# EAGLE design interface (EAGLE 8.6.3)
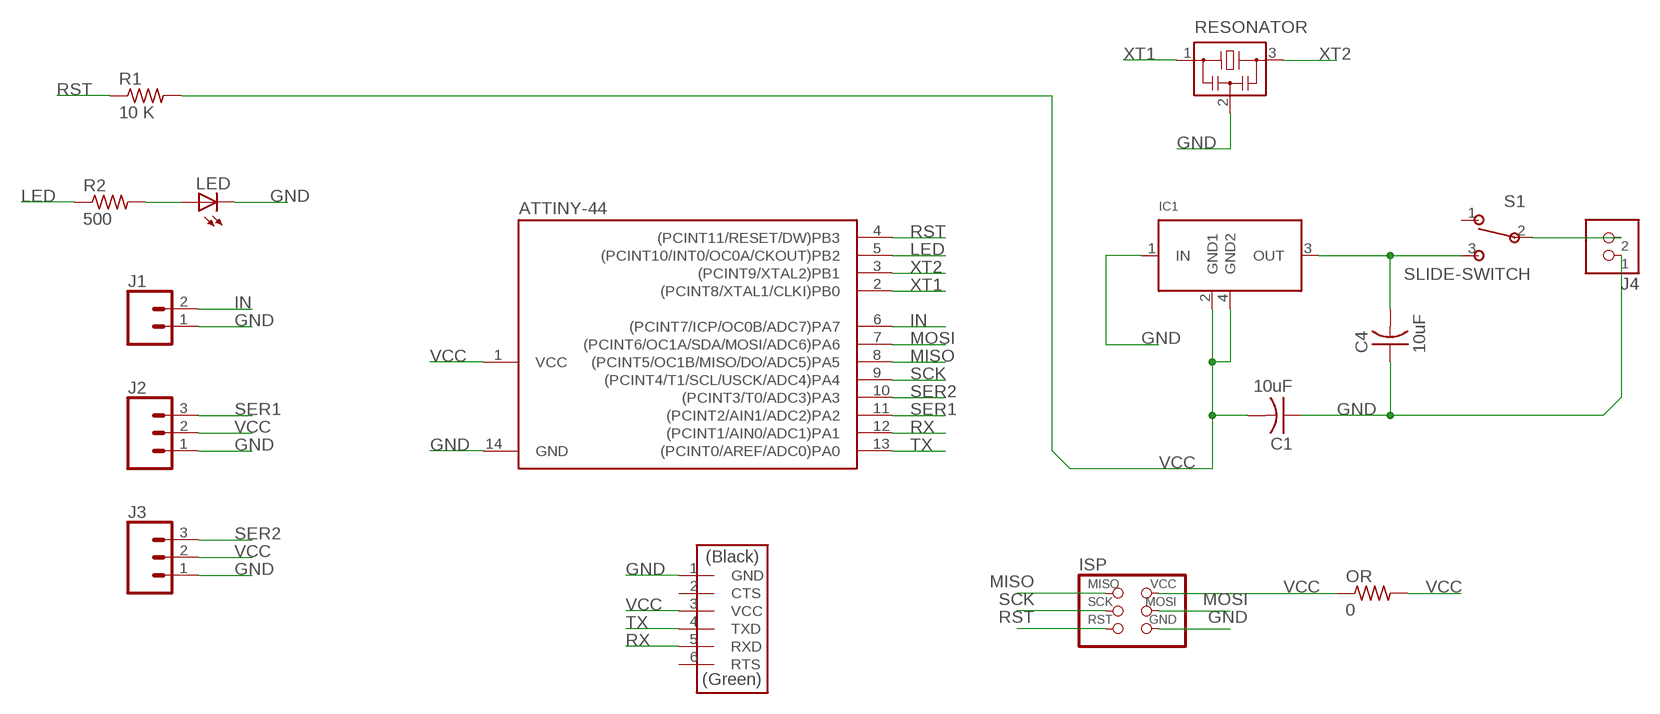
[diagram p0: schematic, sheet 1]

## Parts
ATTINY-44  ATTINY44-SSU  [SOIC14]
C1  10uF  CAP-US1206FAB  [C1206FAB]
C4  10uF  CAP-US1206FAB  [C1206FAB]
IC1  VREG_MULTI  [SOT223]
ISP  AVRISPSMD  [2X03SMD]
J1  CONN_02  [1X02]
J2  CONN_03  [1X03]
J3  CONN_03  [1X03]
J4  TERM-1X02-FABLAB  [ED555DS-2DS]
LED  LEDFAB1206  [LED1206FAB]
OR  0  RES-US1206FAB  [R1206FAB]
R1  10 K  RES-US1206FAB  [R1206FAB]
R2  500  RES-US1206FAB  [R1206FAB]
RESONATOR  RESONATOR  [EFOBM]
S1  SLIDE-SWITCH  [AYZ0102AGRLC]
U$1  FTDI-SMD-HEADER  [1X06SMD]

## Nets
GND: ATTINY-44.14(GND) C1.1 C4.1 IC1.1(IN) ISP.6(GND) J1.1 J2.1 J3.1 J4.1 LED.2(C) RESONATOR.2 U$1.1(GND)
IN: ATTINY-44.6((PCINT7/ICP/OC0B/ADC7)PA7) J1.2
LED: ATTINY-44.5((PCINT10/INT0/OC0A/CKOUT)PB2) R2.1
MISO: ATTINY-44.8((PCINT5/OC1B/MISO/DO/ADC5)PA5) ISP.1(MISO)
MOSI: ATTINY-44.7((PCINT6/OC1A/SDA/MOSI/ADC6)PA6) ISP.4(MOSI)
N$3: C4.2 IC1.3(OUT) S1.3
N$5: J4.2 S1.2
N$6: LED.1(A) R2.2
RST: ATTINY-44.4((PCINT11/RESET/DW)PB3) ISP.5(RST) R1.1
RX: ATTINY-44.12((PCINT1/AIN0/ADC1)PA1) U$1.5(RXD)
SCK: ATTINY-44.9((PCINT4/T1/SCL/USCK/ADC4)PA4) ISP.3(SCK)
SER1: ATTINY-44.11((PCINT2/AIN1/ADC2)PA2) J2.3
SER2: ATTINY-44.10((PCINT3/T0/ADC3)PA3) J3.3
TX: ATTINY-44.13((PCINT0/AREF/ADC0)PA0) U$1.4(TXD)
VCC: ATTINY-44.1(VCC) C1.2 IC1.2(GND1) IC1.4(GND2) ISP.2(VCC) J2.2 J3.2 OR.1 OR.2 R1.2 U$1.3(VCC)
XT1: ATTINY-44.2((PCINT8/XTAL1/CLKI)PB0) RESONATOR.1
XT2: ATTINY-44.3((PCINT9/XTAL2)PB1) RESONATOR.3
Unconnected: S1.1 U$1.2(CTS) U$1.6(RTS)

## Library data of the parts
ATTINY-44 = fab:ATTINY44
C1 C4 = fab:CAP-US
IC1 = m-pad-2.1:VREG_MULTI: standard package voltage regulator (LM2940, LM2937, LM340, UA78M05, etc)
ISP = fab:AVRISP
J1 = SparkFun-Connectors:CONN_02: Multi connection point. Often used as Generic Header-pin footprint for 0.1 inch spaced/style header connections
J2 J3 = SparkFun-Connectors:CONN_03: Multi connection point. Often used as Generic Header-pin footprint for 0.1 inch spaced/style header connections On any of the 0.1 inch spaced packages, you can populate with these: Break Away Headers - Straight (PRT-00116) Break Away Male Headers - Right Angle (PRT-00553) Female Headers (PRT-00115)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; PROD_ID: XXX-00000; VALUE: 455-1750-1-ND
J4 = fab:TERM-1X02: 3.5mm terminal block, 2 positions ED555-2DS as found in the fablab inventory.
LED = fab:LED: LED
OR R1 R2 = fab:RES-US: Resistor (US Symbol)
RESONATOR = fab:RESONATOR
S1 = fab:SLIDE-SWITCH: SMD slide-switch AYZ0102AGRLC as found in the fablab inventory. Includes the mounting holes. Made by Zaerc.
U$1 = fab:FTDI-SMD-HEADER

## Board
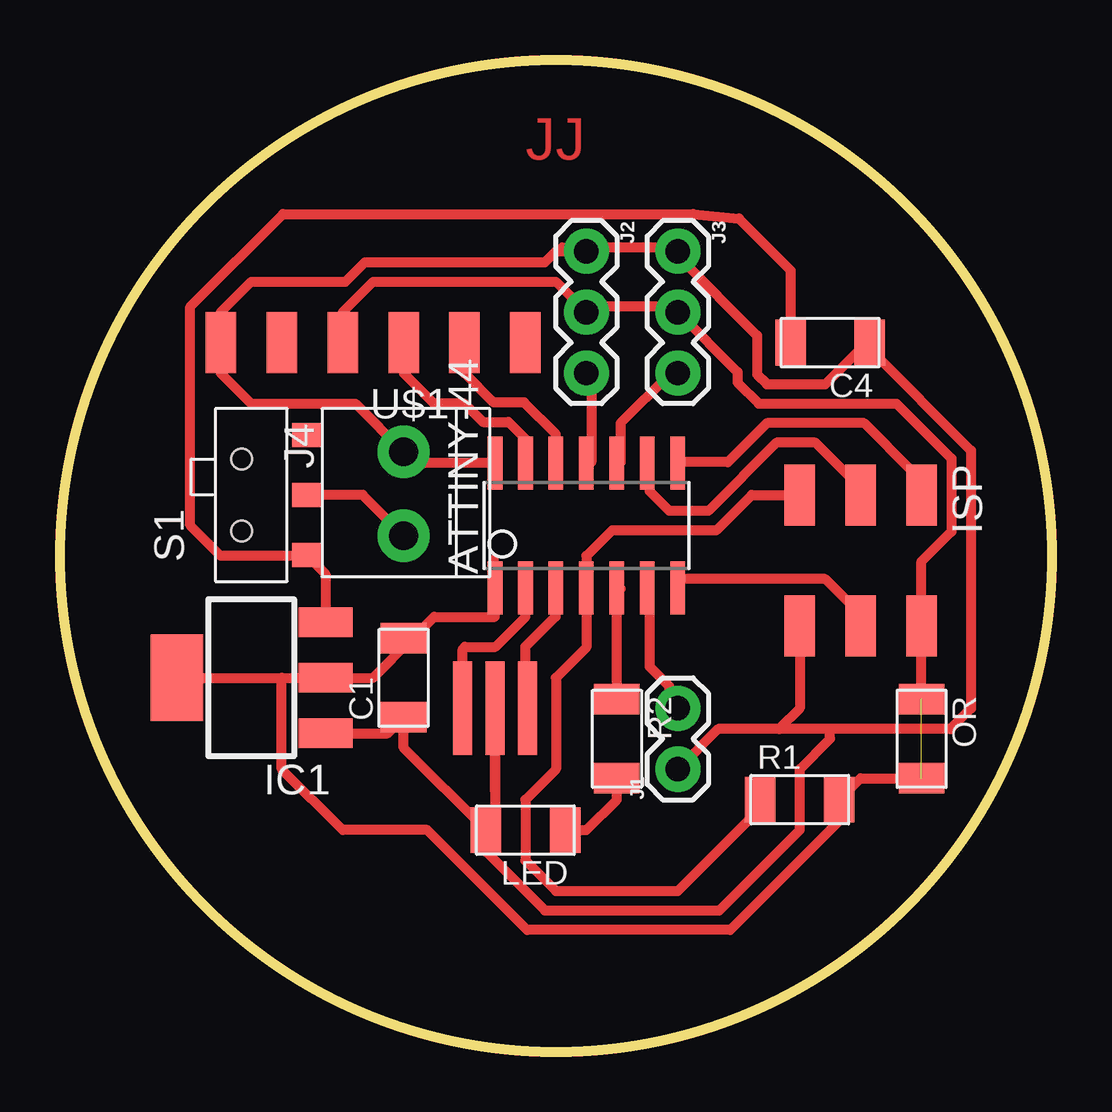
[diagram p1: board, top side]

Size 41.35 x 41.35 mm. Coordinates in mm from the lower left corner, seen from the top.
Outline: circle at 20.67,20.67 radius 20.67
Copper layers (1*16): Top 0.035mm / dielectric 1.5mm / Bottom 0.035mm
Design rules "default *": minimum track width 16mil, minimum drill 0.35mm, track to track 16mil, track to pad 16mil, pad to pad 16mil, via to via 16mil, smd to smd 16mil, copper to edge 16mil, drill to drill 16mil, minimum pad ring 10mil, minimum via ring 8mil, stop-mask expansion 4mil, vias tented up to drill 0mil, thermal gap 10mil

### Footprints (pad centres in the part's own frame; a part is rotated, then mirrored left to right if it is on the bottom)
SOIC14 = smd 0.61 x 2.21: 1 -3.81,-2.603; 2 -2.54,-2.603; 3 -1.27,-2.603; 4 0,-2.603; 5 1.27,-2.603; 6 2.54,-2.603; 7 3.81,-2.603; 8 3.81,2.603; 9 2.54,2.603; 10 1.27,2.603; 11 0,2.603; 12 -1.27,2.603; 13 -2.54,2.603; 14 -3.81,2.603
C1206FAB = smd 1.27 x 1.905: 1 -1.651,0; 2 1.651,0
SOT223 = smd 1.219 x 2.235: 1 -2.311,-3.099; 2 0,-3.099; 3 2.311,-3.099 | smd 3.6 x 2.2: 4 0,3.099
2X03SMD = smd 2.54 x 1.27: 1 -2.54,2.54; 2 2.92,2.54; 3 -2.54,0; 4 2.92,0; 5 -2.54,-2.54; 6 2.92,-2.54
1X02 = drill 1.016 pad 1.88: 1 0,0; 2 2.54,0
1X03 = drill 1.016 pad 1.88: 1 0,0; 2 2.54,0; 3 5.08,0
ED555DS-2DS = drill 1.2 pad 2.184: 1 1.8,0; 2 -1.7,0
LED1206FAB = smd 1.27 x 1.905: 1 -1.651,0; 2 1.651,0
R1206FAB = smd 1.27 x 1.905: 1 -1.651,0; 2 1.651,0
EFOBM = smd 0.8 x 3.9: 1 -1.35,0; 2 0,0; 3 1.35,0
AYZ0102AGRLC = smd 1 x 1.2: 1 2.5,-2.3; 2 0,-2.3; 3 -2.5,-2.3 | hole 0.85: -1.5,0.4; 1.5,0.4
1X06SMD = smd 2.54 x 1.27: 1 0,6.35; 2 0,3.81; 3 0,1.27; 4 0,-1.27; 5 0,-3.81; 6 0,-6.35

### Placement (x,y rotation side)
ATTINY-44  21.94,21.94 0 top
C1  14.32,15.59 90 top
C4  32.1,29.56 180 top
IC1  7.97,15.59 90 top
ISP  33.37,20.67 270 top
J1  25.75,11.78 90 top
J2  21.94,33.37 270 top
J3  25.75,33.37 270 top
J4  14.32,23.21 90 top
LED  19.4,9.24 180 top
OR  35.91,13.05 270 top
R1  30.83,10.51 0 top
R2  23.21,13.05 270 top
RESONATOR  18.13,14.32 0 top
S1  7.97,23.21 90 top
U$1  13.05,29.56 90 top

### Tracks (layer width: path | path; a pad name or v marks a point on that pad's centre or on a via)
GND
  Top 0.406: 30.68,17.68 ISP.6 | 25.81,11.99 J1.1 27.43,13.46 29.97,13.46 | J2.1 22.15,33.53 25.4,33.53 J3.1 25.81,33.12 29.06,29.87 29.06,28.24 29.46,27.84 31.9,27.84 33.53,29.46 C4.1 33.76,29.29 37.97,25.07 37.97,14.31 37.12,13.46 32.1,13.46 | 20.93,33.53 21.74,33.53 J2.1 | 30.68,17.6 ISP.6 | ATTINY-44.14 14.79,24.55 J4.1 12.31,27.02 7.97,27.02 6.7,28.29 U$1.1 6.7,30.83 7.97,32.1 11.91,32.1 12.72,32.92 20.22,32.92 20.67,33.37 J2.1 | IC1.1 13.66,13.28 C1.1 14.32,12.67 LED.2 | 18.13,10.9 RESONATOR.2 18.13,9.63 LED.2 | 32.1,13.46 29.97,13.46 | ISP.6 30.83,14.32 29.97,13.46 | LED.2 17.75,8.36 20.22,5.89 27.48,5.89 30.83,9.24 30.83,11.78 32.1,13.05 32.1,13.46
IN
  Top 0.406: ATTINY-44.6 24.59,19.3 24.59,16.05 25.4,15.24 25.4,14.43 J1.2
LED
  Top 0.406: 23.37,14.83 R2.1 ATTINY-44.5 23.37,19.3
MISO
  Top 0.406: ATTINY-44.8 25.81,24.59 27.84,24.59 29.46,26.21 33.53,26.21 35.56,24.18 35.56,23.37 ISP.1
MOSI
  Top 0.406: ATTINY-44.7 25.81,19.71 31.9,19.71 33.53,18.08 ISP.4
N$3
  Top 0.406: 30.28,29.87 C4.2 30.45,32.58 28.3,34.73 26.4,34.92 9.3,34.92 5.43,31.06 5.43,21.94 6.7,20.67 10.23,20.67 S1.3 11.05,19.94 11.07,19.92 IC1.3
N$5
  Top 0.406: J4.2 12.62,23.21 S1.2
N$6
  Top 0.406: LED.1 21.94,9.24 23.21,10.51 R2.2
RST
  Top 0.406: ISP.5 28.83,23.21 27.36,21.74 23.01,21.74 21.94,20.67 ATTINY-44.4 21.94,16.86 20.67,15.59 20.67,11.78 19.4,10.51 19.4,7.97 20.67,6.7 25.75,6.7 29.18,10.13 R1.1
RX
  Top 0.406: ATTINY-44.12 20.67,25.75 19.35,27.08 18.08,27.08 16.86,28.29 U$1.5
SCK
  Top 0.406: ATTINY-44.9 24.59,24.18 24.59,23.37 25.4,22.55 27.02,22.55 29.87,25.4 31.49,25.4 33.53,23.37 ISP.3
SER1
  Top 0.406: ATTINY-44.11 22.15,24.59 22.15,28.24 J2.3
SER2
  Top 0.406: ATTINY-44.10 23.37,24.59 23.37,26.21 25.4,28.24 J3.3
TX
  Top 0.406: 19.3,24.59 ATTINY-44.13 19.4,25.55 18.69,26.26 17.63,26.26 16.86,27.02 15.59,27.02 14.32,28.29 U$1.4
VCC  (1 unrouted)
  Top 0.406: 21.74,31.09 J2.2 | J2.2 22.15,31.09 25.4,31.09 J3.2 28.24,28.35 28.24,27.91 29.13,27.02 34.87,27.02 37.16,24.74 37.16,21.69 35.91,20.45 ISP.2 OR.1 | 18.08,18.49 18.08,19.3 | 18.08,19.3 ATTINY-44.1 18.08,19.71 18.08,20.52 | OR.2 33.37,11.4 R1.2 32.49,9.63 27.94,5.08 19.47,5.08 15.3,9.24 11.78,9.24 9.24,11.78 9.24,15.59 | U$1.3 11.78,30.83 13.05,32.1 20.67,32.1 J2.2 | C1.2 14.71,17.25 | 14.71,17.25 15.59,18.13 18.13,18.13 18.13,19.25 18.08,19.3 | IC1.4 9.24,15.59 | 9.24,15.59 IC1.2 13.05,15.59 14.71,17.25
XT1
  Top 0.406: 19.3,19.3 ATTINY-44.2 19.4,18.13 18.15,16.88 16.88,16.88 16.78,16.78 RESONATOR.1
XT2
  Top 0.406: RESONATOR.3 19.4,14.4 19.4,16.9 20.66,18.15 20.66,19.33 ATTINY-44.3

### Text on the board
Top: JJ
